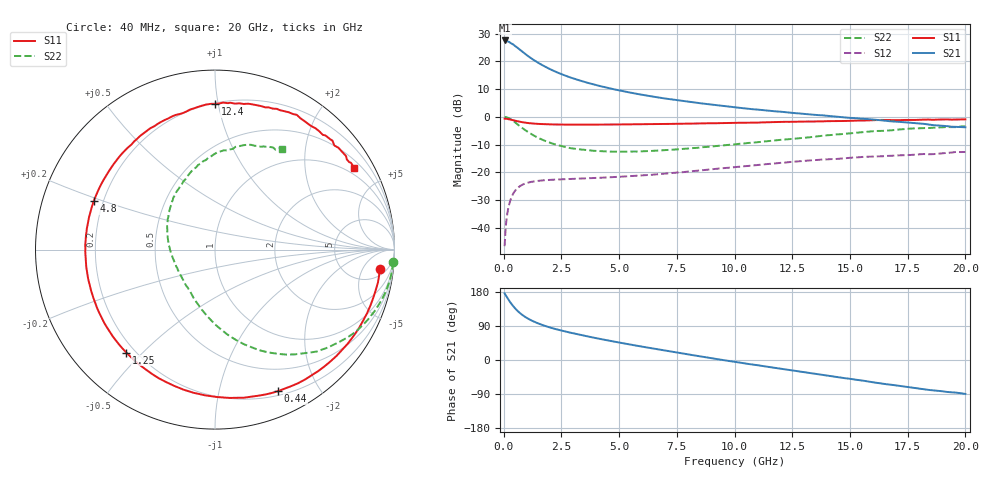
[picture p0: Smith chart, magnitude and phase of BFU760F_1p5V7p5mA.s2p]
! Filename:  P:\Prog\Test\Noise\ATS_data\Testdata_Net\Split files Spar\BFU760F_2W_C1_Bias2_1.5V_5mA_60mA_D.s2p
! Date/Time: Mon 06/Feb/2012 15:06:46
! BFU760_2W_C1_Bias2_1.5V_5mA_60mA_R.s2p
! MDIF S-parameter v. bias file
! BFU760_2W_C1_1.5V_5mA_60mA
! Date/time Fri Mar 18 11:09:37 2011
! VAR V_out= 1.5001
! VAR I_out= 7.5400
! VAR V_in= 0.7678
! VAR I_in= 0.0216
! Device data file deembeded for feedlines and parallel
! Original file: \Split files Spar\BFU760_2W_C1_Bias2_1.5V_5mA_60mA_R.s2p
! Feed-files: PR003V01_101208_Feed1.s2p, PR003V01_101208_Feed2.s2p
! Parallel-file: PR003V01_101208_Par.s2p
# MHz S MA R 50
!  Freq-MHz  S11-mag  S11-arg  S21-mag  S21-arg  S12-mag  S12-arg  S22-mag  S22-arg
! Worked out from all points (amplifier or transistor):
!   167 points, 40 MHz to 20 GHz, reference 50 ohm
!   highest |S21| = 27.5 dB at 50 MHz (marker M1)
!   |S21| within 3 dB of that: start of sweep to 647 MHz
!   unconditionally stable (mu >= 1): 5.608 GHz to 13.55 GHz
!   at 550 MHz: K = 0.10, MSG = 25.7 dB, |S12| = -26.1 dB
!   at 4.2 GHz: K = 0.81, MSG = 16.5 dB, |S12| = -22.0 dB
!   at 20 GHz: K = 0.83, MSG = 4.5 dB, |S12| = -12.7 dB
!   S11 on the Smith chart (normalised r, x): 40 MHz: 8, -12; 440 MHz: 0.24, -1.51; 1.25 GHz: 0.17, -0.45; 4.8 GHz: 0.16, +0.19; 12.4 GHz: 0.21, +0.98; 20 GHz: 0.74, +3.54
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40  0.9272 -6.5  23.78 176.0  0.004652 86.2  0.9961 -4.1
50  0.9251 -8.2  23.79 174.4  0.00554 82.4  0.9948 -5.3
140  0.9185 -22.7  23.22 165.7  0.01611 78.2  0.9772 -14.6
240  0.9019 -38.4  22.31 156.2  0.02662 70.0  0.9373 -24.5
340  0.8829 -52.6  20.91 147.7  0.03562 62.6  0.884 -33.8
440  0.8632 -65.9  19.64 140.1  0.04312 56.1  0.8261 -41.8
600  0.8303 -84.4  17.51 129.5  0.05195 47.4  0.7317 -53.0
700  0.8139 -93.9  16.16 124.1  0.05604 43.0  0.6784 -58.9
850  0.793 -106.4  14.39 117.0  0.06075 37.6  0.6097 -66.6
1050  0.7713 -119.9  12.47 109.3  0.06486 32.2  0.5321 -75.1
1250  0.7571 -130.7  10.91 103.0  0.06778 28.2  0.4736 -82.2
1550  0.7427 -143.1  9.128 95.2  0.07049 23.9  0.407 -91.2
2000  0.7297 -157.0  7.255 85.9  0.07287 19.6  0.3412 -102.7
2600  0.724 -170.3  5.665 76.3  0.07501 16.6  0.2896 -115.1
3400  0.7226 176.4  4.38 65.3  0.07726 14.2  0.2564 -129.0
4800  0.7276 158.3  3.118 48.4  0.08197 13.1  0.2361 -151.1
6800  0.7405 137.7  2.2 26.9  0.09297 12.5  0.2478 -177.6
10200  0.7799 107.8  1.455 -6.7  0.1258 5.7  0.3256 142.7
12400  0.8115 89.8  1.192 -26.8  0.153 -3.4  0.3962 120.4
13400  0.8208 82.3  1.092 -35.6  0.1652 -9.4  0.4348 111.0
16800  0.8724 55.5  0.8273 -65.4  0.1983 -29.6  0.5706 79.9
20000  0.8999 30.4  0.6474 -89.6  0.232 -51.5  0.6757 56.4
